[IBIS Ver]   4.1
[File Name]   f771973xpm.ibs
[File Rev]   1.1
[Date]   DEC 06, 2019
[Source]   File originated at Texas Instruments
[Copyright]   (c) 2012, Texas Instruments Inc.
[Component]   f771973xpm
[Manufacturer] Texas Instruments
[Package]
| Variable   Typ   Min   Max
R_pkg   0.257   0.234   0.294
L_pkg   4.99E-9   4.56E-09   5.76E-09
C_pkg   4.22E-13   3.48E-13   5.29E-13
[Pin]	signal_name	model_name	R_pin	L_pin	C_pin
1	GPIO29	BCPF335585DSHYPBFZ	0.29175	5.7089E-09	4.1442E-13
2	GPIO28	BCF3385DSHYPBFZ_USF	0.27465	5.4118E-09	4.5994E-13
3	XRSN	BQ0491FS_USF	0.26165	5.1378E-09	4.3747E-13
4	VDD	NC	0.25676	5.0126E-09	4.0859E-13
5	VSS	NC	0.25318	4.9188E-09	3.8491E-13
6	A6	ICF33SHYPB_USF	0.28359	5.3331E-09	4.0486E-13
7	C6	ICF33SHYPB_USF	0.27186	5.1029E-09	4.1043E-13
8	A3	ICF33SHYPB_USF	0.2622	4.9365E-09	3.7474E-13
9	A2	ICF33SHYPB_USF	0.24938	4.7865E-09	3.6588E-13
10	A15	ICF33SHYPB_USF	0.24477	4.7119E-09	3.8835E-13
11	C4	ICF33SHYPB_USF	0.2427	4.7374E-09	3.9293E-13
12	A11	ICF33SHYPB_USF	0.24499	4.7879E-09	4.0518E-13
13	A5	ICF33SHYPB_USF	0.24991	4.9002E-09	4.2417E-13
14	A1	ICF33SHYPB_USF	0.25823	5.1095E-09	4.4435E-13
15	A0	ICF33SHYPB_USF	0.27064	5.3367E-09	4.6937E-13
16	VREFHIAC   NC		0.28236	5.6024E-09	4.8293E-13
17	VREFLOAC   NC		0.28165	5.5043E-09	4.7699E-13
18	A12	ICF33SHYPB_USF	0.26312	5.2327E-09	4.6931E-13
19	A7	ICF33SHYPB_USF	0.25068	4.9748E-09	4.4013E-13
20	A8	ICF33SHYPB_USF	0.24125	4.776E-09	4.2229E-13
21	VSSA	NC	0.23697	4.6766E-09	4.6668E-13
22	VDDA	NC	0.23467	4.6004E-09	4.5505E-13
23	A4	ICF33SHYPB_USF	0.23536	4.5689E-09	3.8611E-13
24	C8	ICF33SHYPB_USF	0.2387	4.6274E-09	3.5792E-13
25	A10	ICF33SHYPB_USF	0.24948	4.7621E-09	3.4872E-13
26	VSS	NC	0.24004	4.6485E-09	3.6862E-13
27	VDD	NC	0.24488	4.7634E-09	3.8881E-13
28	VDDSFL	NC	0.24775	4.8744E-09	4.6167E-13
29	GPIO13	BCF3385DSHYPBFZ_USF	0.23751	4.7075E-09	4.0392E-13
30	GPIO12	BCF3385DSHYPBFZ_USF	0.24445	4.9059E-09	4.2591E-13
31	GPIO11	BCF3385DSHYPBFZ_USF	0.2524	5.0619E-09	4.3506E-13
32	GPIO33	BCPF335585DSHYPBFZ	0.28075	5.548E-09	4.1051E-13
33	GPIO16	BCF3385DSHYPBFZ_USF	0.2843	5.5879E-09	4.2432E-13
34	GPIO17	BCF3385DSHYPBFZ_USF	0.2676	5.3024E-09	4.5777E-13
35	GPIO24	BCPF335585DSHYPBFZ	0.26378	5.1765E-09	4.2724E-13
36	TCK	BCF3355DSHYPBFZ_TMS_USF	0.26025	5.0716E-09	4.2027E-13
37	TDO_GPIO37	BCPF335585DSHYPBFZ	0.2566	4.9742E-09	4.1412E-13
38	TMS	BCF3355DSHYPBFZ_TMS_USF	0.24626	4.7978E-09	3.9383E-13
39	TDI_GPIO35	BCF3385DSHYPBFZ_USF	0.24459	4.7103E-09	3.8677E-13
40	GPIO32	BCPF335585DSHYPBFZ	0.25061	4.8085E-09	3.6689E-13
41	GPIO18_X2	BCPF335585DSHYPBFZ	0.25585	4.8744E-09	4.3244E-13
42	GPIO19_X1	BCF3385DSHYPBFZ_USF	0.25951	4.946E-09	4.6364E-13
43	VDDSFL	NC	0.28225	5.0903E-09	5.0424E-13
44	VDD	NC	0.28208	5.1244E-09	5.2952E-13
45	VSS	NC	0.25033	4.8869E-09	4.9543E-13
46	GPIO39	BCF3385DSHYPBFZ_USF	0.25235	5.0001E-09	4.1738E-13
47	GPIO8	BCF3385DSHYPBFZ_USF	0.26444	5.2673E-09	4.426E-13
48	GPIO4	BCF3385DSHYPBFZ_USF	0.2917	5.7116E-09	4.235E-13
49	GPIO3	BCF3385DSHYPBFZ_USF	0.29479	5.765E-09	4.3218E-13
50	GPIO2	BCF3385DSHYPBFZ_USF	0.27638	5.4154E-09	4.6717E-13
51	GPIO1	BCPF335585DSHYPBFZ	0.26947	5.2706E-09	4.4406E-13
52	GPIO0	BCF3385DSHYPBFZ_USF	0.25287	4.9425E-09	4.1354E-13
53	GPIO40	BCF3385DSHYPBFZ_USF	0.25261	4.9194E-09	4.01E-13
54	GPIO23	BCF3385DSHYPBFZ_USF	0.24386	4.7551E-09	3.9602E-13
55	GPIO41	BCF3385DSHYPBFZ_USF	0.23877	4.6355E-09	3.8545E-13
56	GPIO22	BCF3385DSHYPBFZ_USF	0.23699	4.5883E-09	3.5719E-13
57	GPIO7	BCF3385DSHYPBFZ_USF	0.23861	4.622E-09	3.5292E-13
58	VSS	NC	0.24131	4.6594E-09	3.8462E-13
59	VDD	NC	0.27276	4.9291E-09	4.8344E-13
60	VDDSFL	NC	0.24316	4.7926E-09	4.481E-13
61	GPIO5	BCF3385DSHYPBFZ_USF	0.24786	4.8787E-09	4.2176E-13
62	GPIO9	BCF3385DSHYPBFZ_USF	0.25962	5.1027E-09	4.4633E-13
63	GPIO10	BCF3385DSHYPBFZ_USF	0.27403	5.3923E-09	4.5505E-13
64	GPIO6	BCF3385DSHYPBFZ_USF	0.27201	5.402E-09	3.9609E-13
| End of package information
|   Component IQ0440FS_VREGENZ_USF
[Component]   IQ0440FS_VREGENZ_USF
[Manufacturer]   Texas Instruments
[Package]
|  variable   typ   min   max
R_pkg   0   0   0
L_pkg   0   0   0
C_pkg   0   0   0
[Pin]   signal_name   model_name   R_pin   L_pin   C_pin
VSS   VSS   GND
VDDS   VDDS   POWER
PAD   PAD   IQ0440FS_VREGENZ_USF
[Model Selector] IQ0440FS_VREGENZ_USF
VREGENZ_WK_PD_ON_3P3  Cell operated at 3.3(nom)
|VREGENZ_WK_PD_ON_3P3; WEAK_PULLDOWN_ON
VREGENZ_WK_PD_OFF_3P3  Cell operated at 3.3(nom)
|   Component ICF33SHYPB_USF
[Component]   ICF33SHYPB_USF
[Manufacturer]   Texas Instruments
[Package]
|  variable   typ   min   max
R_pkg   0   0   0
L_pkg   0   0   0
C_pkg   0   0   0
[Pin]   signal_name   model_name   R_pin   L_pin   C_pin
VSS   VSS   GND
VDDS   VDDS   POWER
PAD   PAD   ICF33SHYPB_USF
[Model Selector] ICF33SHYPB_USF
ICF_WK_PUPD_OFF_3P3  Cell operated at 3.3(nom)
|ICF_WK_PUPD_OFF_3P3; WEAK_PULL_OFF
ICF_WK_PU_ON_3P3  Cell operated at 3.3(nom)
|ICF_WK_PU_ON_3P3; WEAK_PULLUP_ON
ICF_WK_PD_ON_3P3  Cell operated at 3.3(nom)
|   Component ICF33SHYPB_FS_SFII_CUS
[Component]   ICF33SHYPB_FS_SFII_CUS
[Manufacturer]   Texas Instruments
[Package]
|  variable   typ   min   max
R_pkg   0   0   0
L_pkg   0   0   0
C_pkg   0   0   0
[Pin]   signal_name   model_name   R_pin   L_pin   C_pin
VSS   VSS   GND
VDDS   VDDS   POWER
PAD   PAD   ICF33SHYPB_FS_SFII_CUS
[Model Selector] ICF33SHYPB_FS_SFII_CUS
CUS_WK_PUPD_OFF_3P3  Cell operated at 3.3(nom)
|CUS_WK_PUPD_OFF_3P3; WEAK_PULL_OFF
CUS_WK_PU_ON_3P3  Cell operated at 3.3(nom)
|CUS_WK_PU_ON_3P3; WEAK_PULLUP_ON
CUS_WK_PD_ON_3P3  Cell operated at 3.3(nom)
|   Component BT3308BT5FSHYPB_SFII
[Component]   BT3308BT5FSHYPB_SFII
[Manufacturer]   Texas Instruments
[Package]
|  variable   typ   min   max
R_pkg   0   0   0
L_pkg   0   0   0
C_pkg   0   0   0
[Pin]   signal_name   model_name   R_pin   L_pin   C_pin
VSS   VSS   GND
VDDS   VDDS   POWER
PAD   PAD   BT3308BT5FSHYPB_SFII
[Model Selector] BT3308BT5FSHYPB_SFII
BT_OPEN_DRAIN_6MA_3P3  Cell operated at 3.3(nom)
|BT_OPEN_DRAIN_6MA_3P3
BT_WEAK_PD_ON_3P3  Cell operated at 3.3(nom)
|BT_WEAK_PD_ON_3P3
BT_OPEN_DRAIN_3MA_3P3  Cell operated at 3.3(nom)
|BT_OPEN_DRAIN_3MA_3P3
BT_DRIVER_MODE_6MA_3P3  Cell operated at 3.3(nom)
|BT_DRIVER_MODE_6MA_3P3
BT_DRIVER_MODE_3MA_3P3  Cell operated at 3.3(nom)
|BT_DRIVER_MODE_3MA_3P3
BT_WEAK_PU_ON_3P3  Cell operated at 3.3(nom)
|   Component BQ0491FS_USF
[Component]   BQ0491FS_USF
[Manufacturer]   Texas Instruments
[Package]
|  variable   typ   min   max
R_pkg   0   0   0
L_pkg   0   0   0
C_pkg   0   0   0
[Pin]   signal_name   model_name   R_pin   L_pin   C_pin
VSS   VSS   GND
VDDS   VDDS   POWER
PAD   PAD   BQ0491FS_USF
[Model Selector] BQ0491FS_USF
XRSN_WK_PU_ON_3P3  Cell operated at 3.3(nom)
|XRSN_WK_PU_ON_3P3; WEAK_PULLUP_ON
XRSN_OPEN_DRAIN  Cell operated at 3.3(nom)
|   Component BCPF335585DSHYPBFZ
[Component]   BCPF335585DSHYPBFZ
[Manufacturer]   Texas Instruments
[Package]
|  variable   typ   min   max
R_pkg   0   0   0
L_pkg   0   0   0
C_pkg   0   0   0
[Pin]   signal_name   model_name   R_pin   L_pin   C_pin
VSS   VSS   GND
VDDS   VDDS   POWER
PAD   PAD   BCPF335585DSHYPBFZ
[Model Selector] BCPF335585DSHYPBFZ
BCPF_WK_PU_ON_3P3  Cell operated at 3.3(nom)
|BCPF_WK_PU_ON_3P3; WEAK_PULLUP_ON
BCPF_DRIVER_4MA_3P3  Cell operated at 3.3(nom)
|BCPF_DRIVER_4MA_3P3
BCPF_DRIVER_2MA_3P3  Cell operated at 3.3(nom)
|BCPF_DRIVER_2MA_3P3
BCPF_WK_PD_ON_3P3  Cell operated at 3.3(nom)
|   Component BCF3385DSHYPBFZ_USF
[Component]   BCF3385DSHYPBFZ_USF
[Manufacturer]   Texas Instruments
[Package]
|  variable   typ   min   max
R_pkg   0   0   0
L_pkg   0   0   0
C_pkg   0   0   0
[Pin]   signal_name   model_name   R_pin   L_pin   C_pin
VSS   VSS   GND
VDDS   VDDS   POWER
PAD   PAD   BCF3385DSHYPBFZ_USF
[Model Selector] BCF3385DSHYPBFZ_USF
BCF3385DUSF_WK_PU  Cell operated at 3.3(nom)
| BCF3385DUSF_WK_PU; WEAK_PULLUP_ON
BCF3385DUSF_DRIVER_3P3  Cell operated at 3.3(nom)
|BCF3385DUSF_DRIVER_3P3
BCF3385DUSF_WK_PD  Cell operated at 3.3(nom)
|   Component BCF3385DSHYPBFZ
[Component]   BCF3385DSHYPBFZ
[Manufacturer]   Texas Instruments
[Package]
|  variable   typ   min   max
R_pkg   0   0   0
L_pkg   0   0   0
C_pkg   0   0   0
[Pin]   signal_name   model_name   R_pin   L_pin   C_pin
VSS   VSS   GND
VDDS   VDDS   POWER
PAD   PAD   BCF3385DSHYPBFZ
[Model Selector] BCF3385DSHYPBFZ
BCF3385D_WK_PU_3P3  Cell operated at 3.3(nom)
|BCF3385D_WK_PU_3P3; WEAK_PULLUP_ON
BCF3385D_DRIVER_3P3  Cell operated at 3.3(nom)
|BCF3385D_DRIVER_3P3
BCF3385D_WK_PD_3P3  Cell operated at 3.3(nom)
|   Component BCF3355DSHYPBFZ_TMS_USF
[Component]   BCF3355DSHYPBFZ_TMS_USF
[Manufacturer]   Texas Instruments
[Package]
|  variable   typ   min   max
R_pkg   0   0   0
L_pkg   0   0   0
C_pkg   0   0   0
[Pin]   signal_name   model_name   R_pin   L_pin   C_pin
VSS   VSS   GND
VDDS   VDDS   POWER
PAD   PAD   BCF3355DSHYPBFZ_TMS_USF
[Model Selector] BCF3355DSHYPBFZ_TMS_USF
TMS_WK_PU_ON_3P3  Cell operated at 3.3(nom)
|TMS_WK_PU_ON_3P3; WEAK_PULLUP_ON
TMS_DRIVER_3P3  Cell operated at 3.3(nom)
|TMS_DRIVER_3P3
TMS_WK_PD_ON_3P3  Cell operated at 3.3(nom)
|   Component BCF3335DSHYPBFZ
[Component]   BCF3335DSHYPBFZ
[Manufacturer]   Texas Instruments
[Package]
|  variable   typ   min   max
R_pkg   0   0   0
L_pkg   0   0   0
C_pkg   0   0   0
[Pin]   signal_name   model_name   R_pin   L_pin   C_pin
VSS   VSS   GND
VDDS   VDDS   POWER
PAD   PAD   BCF3335DSHYPBFZ
[Model Selector] BCF3335DSHYPBFZ
BCF3335D_WK_PU_3P3  Cell operated at 3.3(nom)
|BCF3335D_WK_PU_3P3; WEAK_PULLUP_ON
BCF3335D_DRIVER_3P3  Cell operated at 3.3(nom)
|BCF3335D_DRIVER_3P3
BCF3335D_WK_PD_3P3  Cell operated at 3.3(nom)
| Models and submodels in the file (32): VREGENZ_WK_PD_ON_3P3 (Input), VREGENZ_WK_PD_OFF_3P3 (Input), ICF_WK_PUPD_OFF_3P3 (Input), ICF_WK_PU_ON_3P3 (Input), ICF_WK_PD_ON_3P3 (Input), CUS_WK_PUPD_OFF_3P3 (Input), CUS_WK_PU_ON_3P3 (Input), CUS_WK_PD_ON_3P3 (Input), BT_OPEN_DRAIN_6MA_3P3 (I/O_open_drain), BT_WEAK_PD_ON_3P3 (Input), BT_OPEN_DRAIN_3MA_3P3 (I/O_open_drain), BT_DRIVER_MODE_6MA_3P3 (I/O), BT_DRIVER_MODE_3MA_3P3 (I/O), BT_WEAK_PU_ON_3P3 (Input), XRSN_WK_PU_ON_3P3 (Input), XRSN_OPEN_DRAIN (I/O_open_drain), BCPF_WK_PU_ON_3P3 (Input), BCPF_DRIVER_4MA_3P3 (I/O), BCPF_DRIVER_2MA_3P3 (I/O), BCPF_WK_PD_ON_3P3 (Input), BCF3385DUSF_WK_PU (Input), BCF3385DUSF_DRIVER_3P3 (I/O), BCF3385DUSF_WK_PD (Input), BCF3385D_WK_PU_3P3 (Input), BCF3385D_DRIVER_3P3 (I/O), BCF3385D_WK_PD_3P3 (Input), TMS_WK_PU_ON_3P3 (Input), TMS_DRIVER_3P3 (I/O), TMS_WK_PD_ON_3P3 (Input), BCF3335D_WK_PU_3P3 (Input), BCF3335D_DRIVER_3P3 (I/O), BCF3335D_WK_PD_3P3 (Input)
